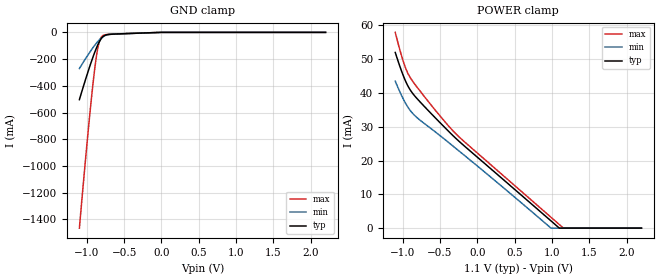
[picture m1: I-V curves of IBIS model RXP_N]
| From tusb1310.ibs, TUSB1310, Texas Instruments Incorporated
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|   RXP_N Input model
[Model]   RXP_N
Model_type   Input
Vinl = 0.35V
Vinh = 0.715V
|   typ   min   max
|   (nom PVT)   (Fast PVT)   (slow PVT)
C_comp   2.352pF   1.988pF   2.902pF
[Voltage Range]   1.1   0.99   1.155
[Temperature Range]   27   105   -40
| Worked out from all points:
|   GND clamp passes 1 mA (typ) near -0.05 V on its own axis
[GND Clamp]
|   Voltage   I(typ)   I(min)   I(max)
-1.1V     -503.3mA   -270.9mA   -1.465A
-1.034V   -381.9mA   -211.2mA   -1.049A
-984.2mV  -294.5mA   -168.2mA   -750.8mA
-942.9mV  -225mA     -134mA     -516.7mA
-901.5mV  -160mA     -101.8mA   -306.1mA
-868.4mV  -113.2mA   -78.33mA   -167.8mA
-843.6mV  -82.41mA   -62.44mA   -92.88mA
-818.8mV  -56.94mA   -48.5mA    -48.05mA
-794mV    -38.04mA   -36.95mA   -27.66mA
-694.7mV  -14.71mA   -15.15mA   -14.99mA
0V        0A         0A         0A
2.2V      0A         0A         0A
[POWER Clamp]
|   Voltage   I(typ)   I(min)   I(max)
-1.1V     51.96mA    43.46mA    57.9mA
-1.042V   48.11mA    40.5mA     53.03mA
-992.5mV  45.12mA    38.19mA    49.32mA
-951.1mV  42.97mA    36.52mA    46.79mA
-909.8mV  41.25mA    35.11mA    44.92mA
-794mV    37.98mA    32.41mA    41.31mA
-421.8mV  29.45mA    25.99mA    31.15mA
-198.5mV  24.77mA    21.98mA    26.05mA
984.2mV   2.206mA    77.67uA    3.283mA
1.1V      0A         0A         1.052mA
1.15V     0A         0A         96.58uA
2.2V      0A         0A         0A
